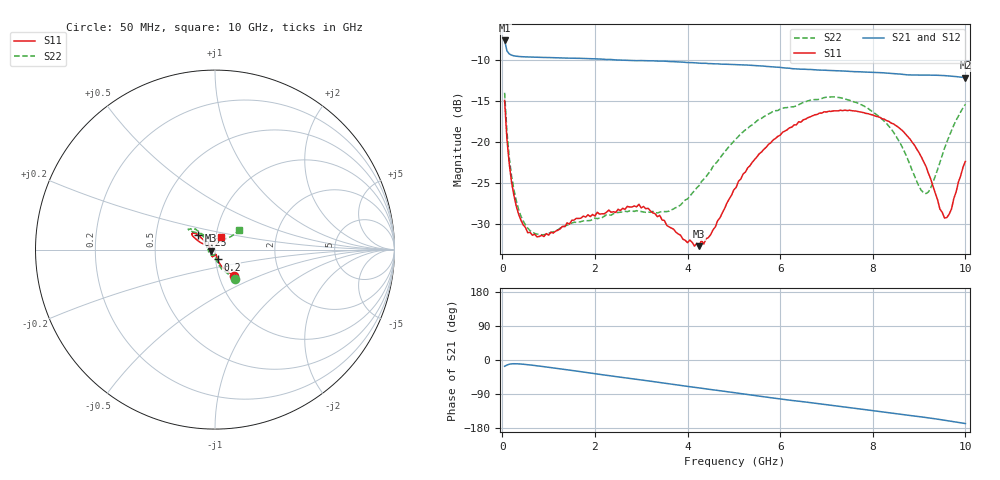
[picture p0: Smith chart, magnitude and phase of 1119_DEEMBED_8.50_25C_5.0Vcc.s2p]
!Hittite Microwave Corp.
!Digital Attenuator/PhaseShifter Rev 1.4.0
!Filename: C:\DATA\DATA\1119_DEEMBED_8.50_25C_5.0Vcc.s2p
!VNA ID: Agilent Technologies,N5224A,MY51441122,A.10.45.03
!Device type:
!2 Port Calibration.
!Temp(C): 25
!Lot Number:
!Serial Number:
!Operator:
!Misc:
!Attenuator:  8.500
# GHZ S DB R 50.0
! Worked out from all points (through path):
!   200 points, 50 MHz to 10 GHz, reference 50 ohm
!   highest |S21| = -7.63 dB at 50 MHz (marker M1); lowest = -12.2 dB at 10 GHz (marker M2)
!   group delay of S21, straight-line fit = 45 ps
!   lowest |S11| = -32.7 dB at 4.25 GHz (marker M3), VSWR 1.05, Z = 47.8 - j0.525 ohm
!   |S11| at or under -10 dB: start of sweep to end of sweep
!   |S22| runs from -31.3 to -14.0 dB; largest |S21 - S12| = 0.00081
!   S11 on the Smith chart (normalised r, x): 50 MHz: 1.17, -0.35; 200 MHz: 1.02, -0.11; 6.25 GHz: 0.82, +0.13; 10 GHz: 1.06, +0.15
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0.05  -14.93 -54.7  -7.63 -16.6  -7.63 -16.6  -14.00 -55.6
0.1  -19.63 -68.3  -8.89 -13.3  -8.89 -13.3  -18.73 -70.9
0.2  -24.89 -75.1  -9.42 -10.2  -9.43 -10.2  -24.12 -81.0
0.4  -29.48 -77.5  -9.60 -10.6  -9.60 -10.6  -29.00 -86.5
0.65  -31.35 -81.0  -9.66 -13.8  -9.66 -13.8  -30.97 -90.7
1.75  -29.02 -103.3  -9.82 -31.8  -9.82 -31.8  -29.60 -108.3
2.95  -27.58 -111.6  -10.08 -51.7  -10.09 -51.8  -28.44 -146.2
3.4  -28.93 -122.5  -10.14 -59.4  -10.15 -59.4  -28.53 -166.5
3.85  -31.34 -140.3  -10.26 -67.2  -10.26 -67.2  -27.66 169.4
4.25  -32.68 -166.3  -10.39 -73.8  -10.41 -73.8  -25.31 149.3
4.5  -31.28 172.1  -10.45 -77.8  -10.47 -77.9  -23.50 140.3
5.05  -25.52 145.1  -10.57 -86.8  -10.59 -86.9  -19.59 131.3
5.55  -21.42 139.7  -10.73 -95.3  -10.75 -95.4  -17.22 132.0
6.25  -18.19 139.2  -11.06 -106.7  -11.08 -106.7  -15.72 135.3
6.7  -16.80 141.1  -11.18 -113.3  -11.19 -113.3  -14.85 140.0
7.65  -16.24 147.1  -11.43 -128.0  -11.44 -128.1  -15.19 143.3
8.35  -17.49 150.0  -11.61 -139.5  -11.62 -139.5  -18.09 133.3
8.75  -19.26 152.4  -11.82 -145.8  -11.81 -145.8  -22.02 119.4
9.15  -22.98 154.1  -11.85 -151.8  -11.86 -151.8  -26.27 82.8
9.55  -29.26 117.2  -11.91 -159.0  -11.92 -159.0  -20.75 43.0
9.7  -28.16 87.2  -11.98 -161.9  -11.99 -161.9  -18.60 39.1
10  -22.36 65.3  -12.16 -167.7  -12.17 -167.7  -15.40 39.1
